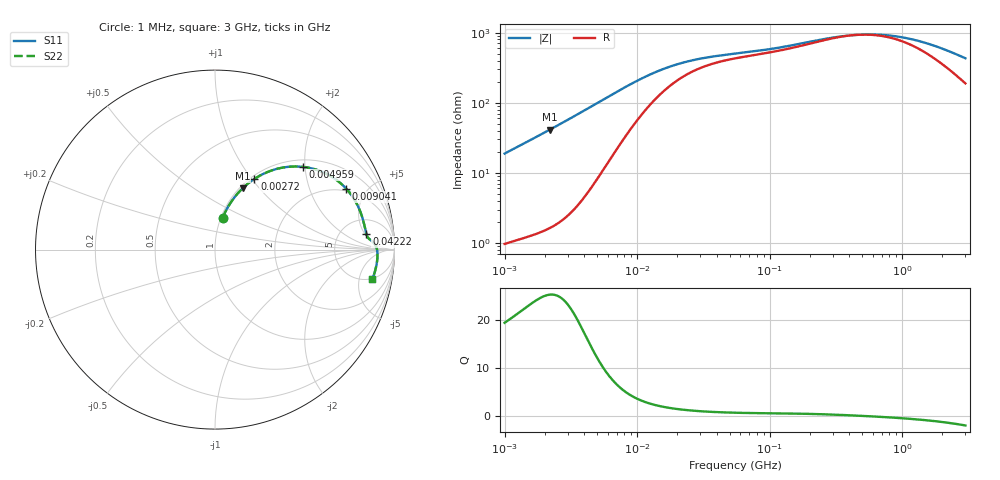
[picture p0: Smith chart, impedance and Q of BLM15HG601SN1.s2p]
! BLM15HG601SN1
# Hz S RI R 50
!Freq.(Hz) S11(Real) S11(Imag) S21(Real) S21(Imag) S12(Real) S12(Imag) S22(Real) S22(Imag)
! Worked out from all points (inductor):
!   401 points, 1 MHz to 3 GHz, reference 50 ohm
!   read as one part in series: L = 2.99 uH near 1.041 MHz
!   highest Q = 25.2 at 2.183 MHz (marker M1), where L = 2.99 uH
!   self-resonance near 455 MHz
!   S11 on the Smith chart (normalised r, x): 1 MHz: 1.02, +0.38; 2.72 MHz: 1.04, +1.03; 4.959 MHz: 1.16, +1.96; 9.041 MHz: 1.87, +3.62; 42.22 MHz: 9, +5; 3 GHz: 4.77, -7.75
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1000000  0.0428 0.1783  0.9572 -0.1783  0.9572 -0.1783  0.0428 0.1783
1522470  0.085 0.258  0.915 -0.258  0.915 -0.258  0.085 0.258
2182827  0.1542 0.3419  0.8458 -0.3419  0.8458 -0.3419  0.1542 0.3419
2720446  0.2196 0.394  0.7804 -0.394  0.7804 -0.394  0.2196 0.394
3823119  0.3611 0.4537  0.6389 -0.4537  0.6389 -0.4537  0.3611 0.4537
4959344  0.4912 0.4607  0.5088 -0.4607  0.5088 -0.4607  0.4912 0.4607
6831390  0.6397 0.4124  0.3603 -0.4124  0.3603 -0.4124  0.6397 0.4124
9040831  0.7312 0.3392  0.2688 -0.3392  0.2688 -0.3392  0.7312 0.3392
1.126754e7  0.776 0.2798  0.224 -0.2798  0.224 -0.2798  0.776 0.2798
1.461624e7  0.8067 0.2188  0.1933 -0.2188  0.1933 -0.2188  0.8067 0.2188
2.41077e7  0.832 0.1371  0.168 -0.1371  0.168 -0.1371  0.832 0.1371
4.22235e7  0.8431 0.0879  0.1569 -0.0879  0.1569 -0.0879  0.8431 0.0879
5.477226e7  0.8476 0.0748  0.1524 -0.0748  0.1524 -0.0748  0.8476 0.0748
1.081723e8  0.8649 0.0545  0.1351 -0.0545  0.1351 -0.0545  0.8649 0.0545
2.094008e8  0.8871 0.0345  0.1129 -0.0345  0.1129 -0.0345  0.8871 0.0345
4.304467e8  0.9022 0.00274  0.0978 -0.00274  0.0978 -0.00274  0.9022 0.00274
5.929311e8  0.9047 -0.0137  0.0953 0.0137  0.0953 0.0137  0.9047 -0.0137
8.005644e8  0.9054 -0.0311  0.0946 0.0311  0.0946 0.0311  0.9054 -0.0311
1.080907e9  0.9043 -0.0514  0.0957 0.0514  0.0957 0.0514  0.9043 -0.0514
1.45942e9  0.9012 -0.0764  0.0988 0.0764  0.0988 0.0764  0.9012 -0.0764
1.970482e9  0.8949 -0.1077  0.1051 0.1077  0.1051 0.1077  0.8949 -0.1077
3e9  0.8763 -0.166  0.1237 0.166  0.1237 0.166  0.8763 -0.166
